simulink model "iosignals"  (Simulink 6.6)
settings: Solver=ode23s  StartTime=0.0  StopTime=400  RelTol=1e-6
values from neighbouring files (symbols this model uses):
  design = []    [designpid.m]
libraries: cstextras x2, simulink x1, cstblocks x1

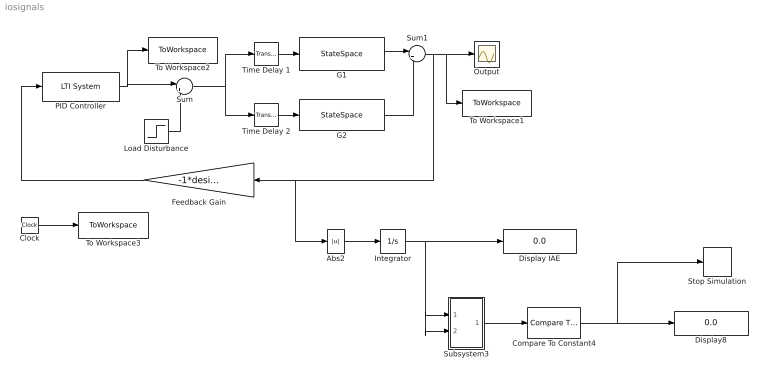
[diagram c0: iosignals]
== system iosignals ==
  Abs2 : Abs
  Clock : Clock
  Compare To Constant4 : simulink/Logic and Bit Operations/Compare To Constant  SystemSampleTime=-1  relop=<=  const=0.001  LogicOutDataTypeMode=boolean  ZeroCross=off
  Display IAE : Display
  Display8 : Display
  Feedback Gain : Gain  Orientation=left  Gain=-1*design.sim.sgn
  G1 : StateSpace  A=design.sim.G1a  B=design.sim.G1b  C=design.sim.G1c  D=design.sim.G1d
  G2 : StateSpace  A=design.sim.G2a  B=design.sim.G2b  C=design.sim.G2c  D=design.sim.G2d
  Integrator : Integrator
  Load Disturbance : Step  Time=0  SampleTime=0
  Output : Scope
  PID Controller : cstblocks/LTI System  SystemSampleTime=-1  sys=design.PID.Grfinal  IC=[]
  Stop Simulation : Stop
  Subsystem3 : Subsystem
  Sum : Sum  Inputs=|++
  Sum1 : Sum  Inputs=|++
  Time Delay 1 : cstextras/Transport Delay (masked)  Tag=InputDelayBlock  SystemSampleTime=-1  Td=design.sim.L1  u0=0  bufsize=100000
  Time Delay 2 : cstextras/Transport Delay (masked)  Tag=InputDelayBlock  SystemSampleTime=-1  Td=design.sim.L2  u0=0  bufsize=100000
  To Workspace1 : ToWorkspace  VariableName=outputsignal  SampleTime=-1  SaveFormat=Array
  To Workspace2 : ToWorkspace  VariableName=controlsignal  SampleTime=-1  SaveFormat=Array
  To Workspace3 : ToWorkspace  VariableName=timesignal  SampleTime=-1  SaveFormat=Array
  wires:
  Sum/1 -> Time Delay 1/1, Time Delay 2/1
  PID Controller/1 -> Sum/1, To Workspace2/1
  Load Disturbance/1 -> Sum/2
  Time Delay 1/1 -> G1/1
  G1/1 -> Sum1/1
  Time Delay 2/1 -> G2/1
  Sum1/1 -> Feedback Gain/1, Abs2/1, Output/1, To Workspace1/1
  Feedback Gain/1 -> PID Controller/1
  G2/1 -> Sum1/2
  Integrator/1 -> Display IAE/1, Subsystem3/2(In2), Subsystem3/1(In1)
  Subsystem3/1(Out1) -> Compare To Constant4/1
  Compare To Constant4/1 -> Display8/1, Stop Simulation/1
  Abs2/1 -> Integrator/1
  Clock/1 -> To Workspace3/1

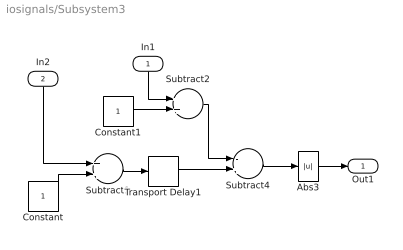
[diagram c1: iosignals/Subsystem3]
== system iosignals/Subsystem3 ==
  In1 : Inport  Orientation=down
  In2 : Inport  Orientation=down  Port=2
  Abs3 : Abs  ZeroCross=off
  Constant : Constant
  Constant1 : Constant
  Subtract1 : Sum  OutScaling=2^-10
  Subtract2 : Sum  OutScaling=2^-10
  Subtract4 : Sum  Inputs=-+  OutScaling=2^-10
  Transport Delay1 : TransportDelay  DelayTime=25  BufferSize=10000
  Out1 : Outport
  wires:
  Abs3/1 -> Out1/1
  Subtract4/1 -> Abs3/1
  Transport Delay1/1 -> Subtract4/2
  Constant/1 -> Subtract1/2
  In2/1 -> Subtract1/1
  Subtract1/1 -> Transport Delay1/1
  Constant1/1 -> Subtract2/2
  Subtract2/1 -> Subtract4/1
  In1/1 -> Subtract2/1
